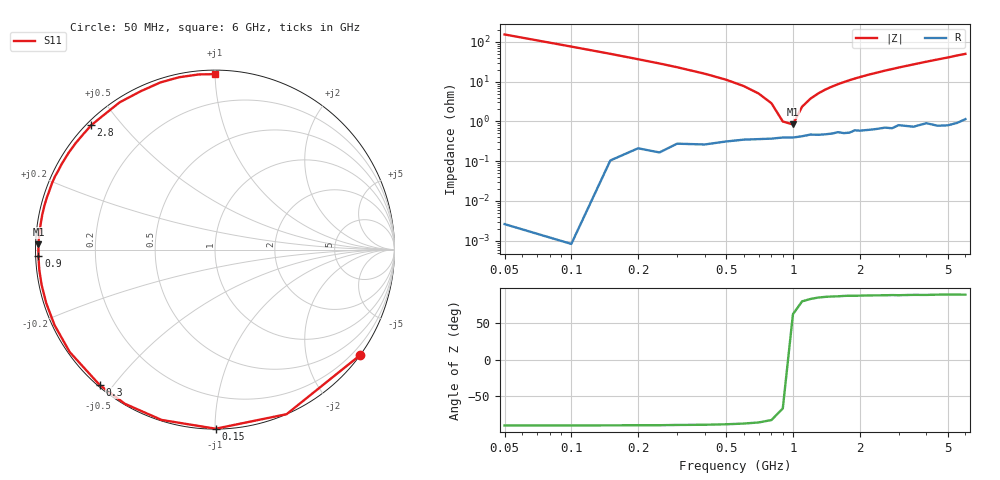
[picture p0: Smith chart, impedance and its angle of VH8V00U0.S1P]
! Infineon Technologies  Discrete & RF Semiconductors
! BB 814
! Si Tuning Diode in SOT23
! VR = 8 V
! S-Parameters:  July  1999
# GHz  S  MA  R  50
!  f  S11
! GHz  MAG  ANG
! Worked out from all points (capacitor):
!   34 points, 50 MHz to 6 GHz, reference 50 ohm
!   read as one part to ground: C = 20.6 pF near 50 MHz
!   lowest |Z| = 840 mohm at 1 GHz (marker M1)
!   series resonance near 955.3 MHz, so ESL is about 1.3 nH
!   S11 on the Smith chart (normalised r, x): 50 MHz: 0.00, -3.08; 150 MHz: 0.00, -1.00; 300 MHz: 0.01, -0.46; 900 MHz: 0.01, -0.02; 2.8 GHz: 0.01, +0.42; 6 GHz: 0.02, +1.00
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0.05  1 -36.0
0.1  1 -66.5
0.15  0.9979 -89.8
0.2  0.9945 -107.4
0.25  0.995 -120.3
0.3  0.9909 -130.4
0.4  0.9905 -144.8
0.5  0.9881 -154.8
0.6  0.9865 -162.4
0.7  0.9859 -168.5
0.8  0.9854 -173.5
0.9  0.9843 -177.9
1  0.9844 178.3
1.1  0.9832 174.7
1.3  0.9819 168.5
1.6  0.9793 160.3
1.8  0.9802 155.4
2  0.9782 150.9
2.2  0.9777 146.5
2.4  0.9769 142.6
2.6  0.9758 138.5
2.8  0.9772 134.9
3.5  0.9775 122.9
4  0.9746 115.1
4.5  0.9798 108.1
5  0.9809 101.8
5.5  0.9802 95.3
6  0.9774 90.0
